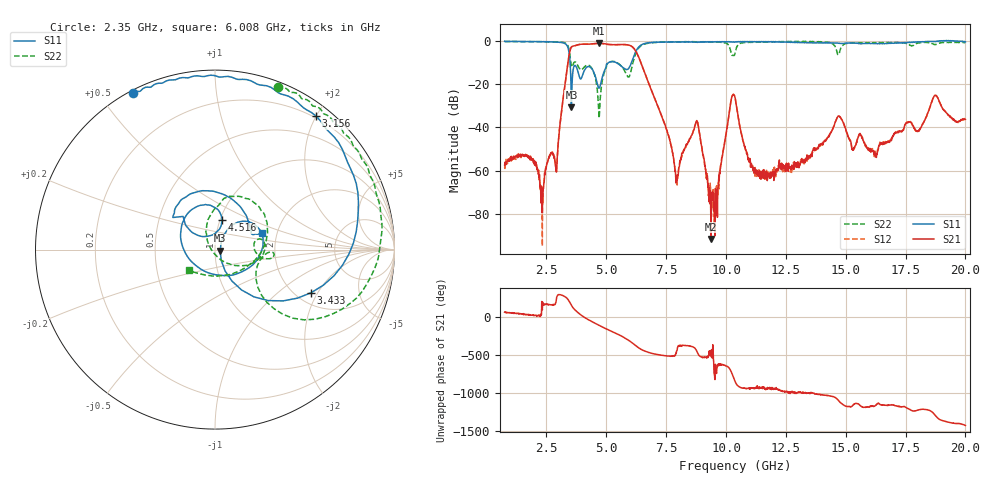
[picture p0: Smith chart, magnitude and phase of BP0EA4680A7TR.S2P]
! s2p File.  Ports: 1,3
# MHz S DB R 50
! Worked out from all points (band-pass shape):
!   1601 points, 750 MHz to 20 GHz, reference 50 ohm
!   highest |S21| = -0.93 dB at 4.708 GHz (marker M1); lowest = -91.7 dB at 9.376 GHz (marker M2)
!   |S21| within 3 dB of the highest: 3.491 GHz to 6.193 GHz (2.702 GHz wide, 55.8 % of centre)
!   lowest |S11| = -30.7 dB at 3.541 GHz (marker M3), VSWR 1.06, Z = 52.9 - j0.672 ohm
!   |S11| at or under -10 dB: 3.485 GHz to 5.076 GHz (1.591 GHz wide, 37.2 % of centre); 5.428 GHz to 6.045 GHz (616.5 MHz wide, 10.7 % of centre)
!   |S22| runs from -35.7 to 0.0 dB; largest |S21 - S12| = 0.0081
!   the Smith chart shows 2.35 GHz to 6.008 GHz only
!   S11 on the Smith chart (normalised r, x): 2.35 GHz: 0.01, +0.60; 3.156 GHz: 0.17, +2.00; 3.433 GHz: 2.40, -1.76; 4.516 GHz: 1.02, +0.34; 6.008 GHz: 1.68, +0.33
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750  0.02 165.4  -57.50 66.0  -58.27 70.7  -0.16 149.6
2350.16  -0.14 117.8  -71.27 158.5  -74.77 -177.1  -0.24 69.0
3156.25  -0.60 52.8  -29.75 -72.6  -29.74 -72.1  -0.45 14.7
3432.97  -4.62 -24.1  -7.13 -144.0  -7.16 -143.8  -3.37 -34.9
3541.25  -30.67 -12.5  -2.67 154.6  -2.66 154.5  -11.66 -29.1
3962.34  -17.04 -144.3  -1.32 23.8  -1.33 23.7  -13.20 6.6
4515.78  -15.50 76.5  -1.07 -77.4  -1.07 -77.6  -15.87 -33.8
4708.28  -21.58 115.0  -0.93 -109.1  -0.95 -109.1  -34.36 -174.2
5309.84  -9.47 103.6  -1.56 162.2  -1.58 162.4  -9.44 41.0
6007.66  -11.07 19.0  -2.00 39.9  -2.01 39.8  -14.69 -142.0
6464.84  -1.69 -49.2  -10.53 -64.5  -10.55 -64.3  -1.91 77.5
7174.69  -0.38 -109.5  -30.75 -132.7  -30.83 -131.9  -0.45 6.5
7944.69  -0.33 -142.9  -65.08 -80.0  -65.91 -83.0  -0.23 -22.6
8798.91  -0.50 -177.7  -37.11 -100.8  -37.03 -99.7  -0.27 -39.1
9376.41  -0.24 163.3  -91.73 -73.9  -71.46 -133.4  -0.25 -51.7
10375  -0.23 144.3  -26.02 -119.2  -26.03 -120.0  -5.71 -56.6
11337.5  -0.10 131.0  -62.02 155.5  -62.37 152.3  -0.43 -111.7
13587.34  -0.73 60.0  -53.50 88.4  -51.51 87.5  -0.15 -137.5
14706.25  -0.88 6.2  -34.61 -16.8  -34.75 -16.8  -6.10 -138.0
16799.69  -0.89 -93.8  -46.76 -68.8  -46.68 -75.2  -0.56 124.2
18736.72  -0.14 -143.6  -25.12 152.8  -25.05 153.1  -1.49 102.2
20000  -0.24 164.9  -36.27 19.2  -35.83 19.8  -0.64 59.0
